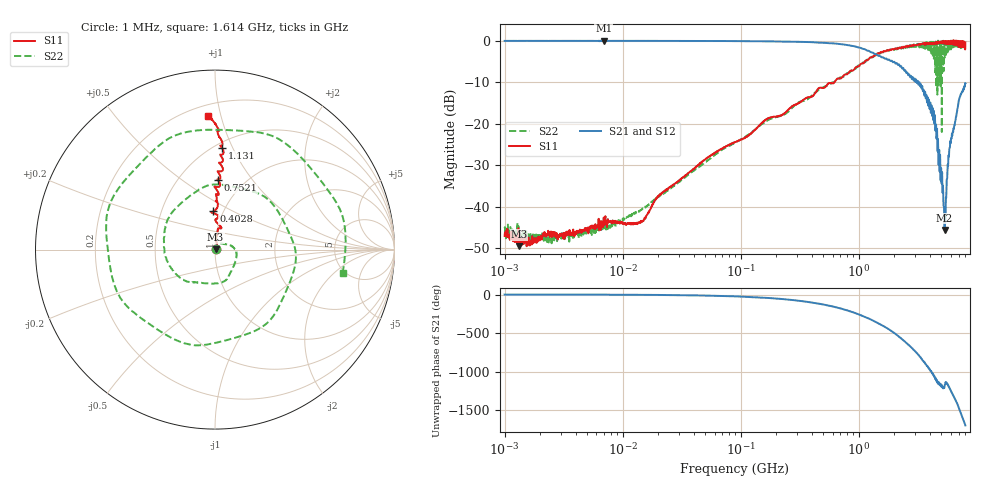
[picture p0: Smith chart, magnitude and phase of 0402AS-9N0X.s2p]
!s-Parameter Generated by FASTRON Sdn. Bhd.
!FASTRON P/N : 0402AS-9N0X
!Keysight Technologies: E5071C_MY46733604_B.14.02
!Date: Mon Dec 01 10:28:47 2025
!Version  :Rev00  Mon Dec 01 10:28:47 2025
!Data & Calibration Information:
!Freq  S11:SOLT2(ON)  S21:SOLT2(ON)  S12:SOLT2(ON)  S22:SOLT2(ON)
!PortZ  Port1:50+j0  Port2:50+j0
!When reading reference impedance value at option line is always used.
! Remarks : This data is being provided solely for informational purposes.
# Hz S dB R 50
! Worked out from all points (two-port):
!   1601 points, 1 MHz to 8 GHz, reference 50 ohm
!   highest |S21| = 0.03 dB at 6.912 MHz (marker M1); lowest = -45.6 dB at 5.332 GHz (marker M2)
!   |S21| within 3 dB of the highest: start of sweep to 1.331 GHz
!   lowest |S11| = -49.5 dB at 1.323 MHz (marker M3), VSWR 1.01, Z = 50.3 + j0.113 ohm
!   |S11| at or under -10 dB: start of sweep to 621.7 MHz
!   |S22| runs from -48.8 to 0.0 dB; largest |S21 - S12| = 0.017
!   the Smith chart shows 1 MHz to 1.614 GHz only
!   S11 on the Smith chart (normalised r, x): 1 MHz: 1.01, +0.00; 402.8 MHz: 0.90, +0.40; 752.1 MHz: 0.76, +0.69; 1.131 GHz: 0.54, +0.91; 1.614 GHz: 0.28, +0.91
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1000000  -47.00 17.1  -0.06 -0.3  -0.04 -0.3  -45.20 18.1
1323440  -49.50 19.6  -0.04 -0.3  -0.04 -0.3  -46.50 9.4
4479405  -45.90 36.9  -0.05 -1.2  -0.04 -1.2  -46.80 38.3
6911657  -42.60 20.8  0.03 -2.1  0.03 -2.2  -43.30 29.7
2.00676e7  -37.50 55.0  -0.05 -5.3  -0.05 -5.3  -37.60 66.9
8.994653e7  -24.40 87.0  -0.10 -23.6  -0.09 -23.6  -24.60 31.7
4.006501e8  -13.50 92.9  -0.36 -104.0  -0.35 -104.0  -13.20 -123.0
4.02787e8  -13.40 92.4  -0.36 -104.0  -0.36 -104.0  -13.20 -124.0
7.521334e8  -8.25 87.5  -0.93 166.0  -0.92 166.0  -8.58 65.2
1.131415e9  -4.91 86.1  -2.10 69.0  -2.10 68.9  -5.17 -130.0
1.411421e9  -3.32 88.9  -3.29 0.7  -3.28 0.6  -3.51 89.4
1.613809e9  -2.58 92.9  -4.05 -47.1  -4.05 -47.2  -2.81 -10.3
1.7949e9  -2.34 95.7  -4.54 -89.6  -4.55 -89.7  -2.43 -97.2
2.135779e9  -1.83 101.0  -5.78 -173.0  -5.77 -173.0  -1.75 92.8
2.501569e9  -1.34 107.0  -7.46 97.7  -7.44 97.7  -1.62 -95.0
2.868376e9  -1.19 115.0  -8.78 16.0  -8.74 15.8  -1.52 93.8
3.223742e9  -0.94 122.0  -10.50 -65.4  -10.50 -65.7  -0.75 -75.0
3.588581e9  -0.62 135.0  -13.20 -158.0  -13.20 -159.0  -0.55 82.9
3.95342e9  -0.64 136.0  -15.10 112.0  -15.10 112.0  -2.27 -103.0
4.296652e9  -0.65 143.0  -18.20 44.1  -18.30 43.5  -0.28 120.0
5.33235e9  -0.25 175.0  -45.60 -103.0  -45.70 -105.0  -3.05 35.6
8e9  -0.46 -98.6  -10.30 104.0  -10.40 104.0  -2.01 143.0
